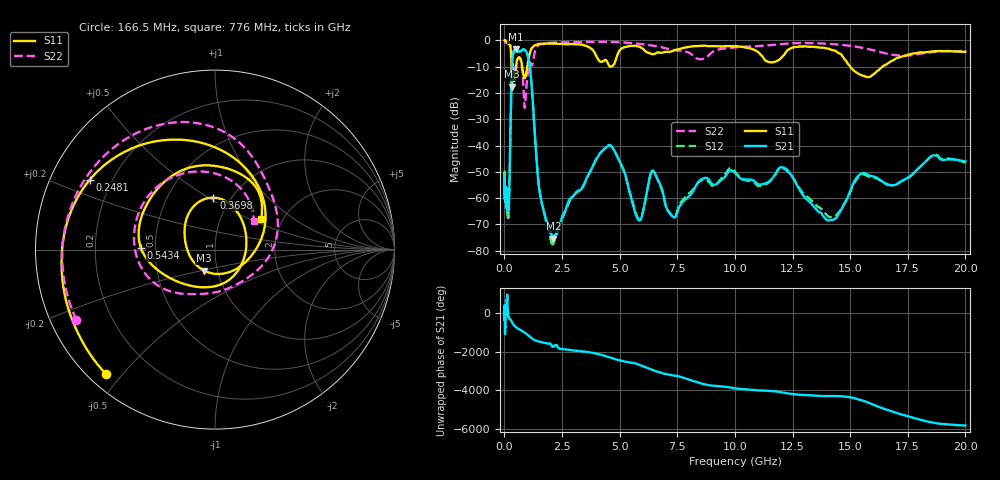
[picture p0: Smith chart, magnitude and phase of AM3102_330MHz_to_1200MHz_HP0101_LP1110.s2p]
! Date/Time: Tue, Sep 11, 2018 5:14 PM
! Network Analyzer: Agilent Technologies E8362B Rev: A.07.50.63
! Sweep from 0.010 to 20.000 GHz, 1601 Points, Sweep Type: LOG
! Power Supply: 4.949 V, 0.001 A
# Hz S DB R 50
!freq MagS11 AngS11 MagS21 AngS21 MagS12 AngS12 MagS22 AngS22
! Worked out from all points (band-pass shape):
!   1601 points, 10 MHz to 20 GHz, reference 50 ohm
!   highest |S21| = -3.35 dB at 482.5 MHz (marker M1); lowest = -75.5 dB at 2.124 GHz (marker M2)
!   |S21| within 3 dB of the highest: 357 MHz to 1.031 GHz (674.2 MHz wide, 97.1 % of centre)
!   lowest |S11| = -17.6 dB at 331.5 MHz (marker M3), VSWR 1.30, Z = 43.1 - j10.3 ohm
!   |S11| at or under -10 dB: 309.5 MHz to 509.3 MHz (199.8 MHz wide, 48.8 % of centre); 772.6 MHz to 988.3 MHz (215.7 MHz wide, 24.5 % of centre); 15.01 GHz to 16.4 GHz (1.399 GHz wide, 8.91 % of centre)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
!   |S22| runs from -25.7 to -0.3 dB; largest |S21 - S12| = 0.012
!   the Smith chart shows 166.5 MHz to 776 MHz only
!   S11 on the Smith chart (normalised r, x): 166.5 MHz: 0.05, -0.45; 248.1 MHz: 0.12, +0.26; 369.8 MHz: 0.83, +0.53; 543.4 MHz: 0.42, +0.01; 776 MHz: 1.56, +0.58
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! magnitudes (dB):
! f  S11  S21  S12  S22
! 10 MHz  0.0  -52.5  -49.4  -0.3
! 35.55 MHz  0.0  -59.0  -59.2  -0.6
! 126.4 MHz  -0.4  -64.3  -61.1  -1.1
! 166.5 MHz  -0.7  -63.3  -65.5  -1.2
! 248.1 MHz  -2.0  -41.8  -41.7  -1.8
! 331.5 MHz  -17.6  -9.1  -9.1  -5.7
! 369.8 MHz  -10.8  -5.6  -5.7  -8.7
! 447.2 MHz  -14.6  -3.5  -3.5  -12.7
! 482.5 MHz  -12.5  -3.4  -3.4  -11.3
! 543.4 MHz  -7.7  -3.8  -3.9  -7.8
! 776 MHz  -10.2  -3.6  -3.6  -11.4
! 882.2 MHz  -14.4  -3.6  -3.6  -25.7
! 1.108 GHz  -4.7  -10.4  -10.4  -8.4
! 1.59 GHz  -1.4  -60.5  -60.7  -1.4
! 2.124 GHz  -1.2  -75.5  -77.3  -0.8
! 4.479 GHz  -8.4  -40.2  -40.0  -0.5
! 5.652 GHz  -2.1  -64.9  -64.3  -1.1
! 6.487 GHz  -5.2  -49.9  -50.1  -2.0
! 7.305 GHz  -4.0  -67.1  -67.0  -3.6
! 12.09 GHz  -5.9  -48.3  -48.6  -1.3
! 14.07 GHz  -3.2  -68.5  -67.0  -1.3
! 20 GHz  -4.3  -46.0  -46.5  -4.2
